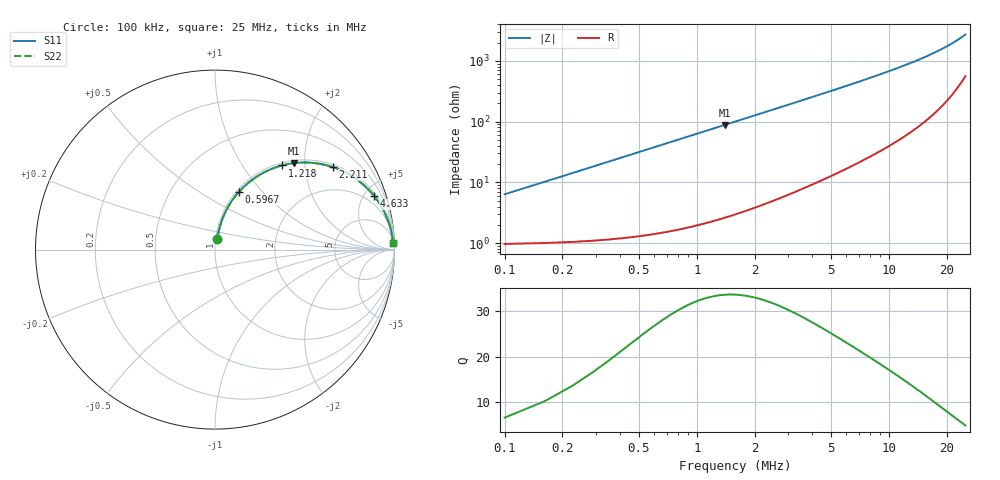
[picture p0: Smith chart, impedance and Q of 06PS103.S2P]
! Coilcraft 0603PS-103 Power Chip Inductor
! 19 February 2003
# MHZ S MA R 50
!Freq  MagS11  AngS11  MagS21  AngS21  MagS12  AngS12  MagS22  AngS22
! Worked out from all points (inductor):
!   403 points, 100 kHz to 25 MHz, reference 50 ohm
!   read as one part in series: L = 10 uH near 224.2 kHz
!   highest Q = 33.7 at 1.404 MHz (marker M1), where L = 10 uH
!   S11 on the Smith chart (normalised r, x): 100 kHz: 1.02, +0.13; 596.7 kHz: 1.03, +0.75; 1.218 MHz: 1.05, +1.53; 2.211 MHz: 1.09, +2.79; 4.633 MHz: 1.23, +5.90; 25 MHz: 12, +53
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0.1  0.06284 77.7  0.9885 -3.6  0.9885 -3.6  0.06284 77.7
0.16209  0.1008 78.6  0.9851 -5.8  0.9851 -5.8  0.1008 78.6
0.28627  0.1755 76.4  0.9739 -10.1  0.9739 -10.1  0.1755 76.4
0.34836  0.2118 74.8  0.9663 -12.2  0.9663 -12.2  0.2118 74.8
0.47254  0.2816 71.2  0.9476 -16.3  0.9476 -16.3  0.2816 71.2
0.59672  0.3471 67.6  0.925 -20.3  0.925 -20.3  0.3471 67.6
0.84508  0.4631 60.6  0.8714 -27.6  0.8714 -27.6  0.4631 60.6
1.03135  0.5367 55.8  0.8274 -32.4  0.8274 -32.4  0.5367 55.8
1.21762  0.5995 51.5  0.7826 -36.8  0.7826 -36.8  0.5995 51.5
1.40389  0.6525 47.6  0.7387 -40.7  0.7387 -40.7  0.6525 47.6
1.77643  0.7347 41.0  0.6568 -47.3  0.6568 -47.3  0.7347 41.0
2.21106  0.801 35.1  0.5746 -53.2  0.5746 -53.2  0.801 35.1
2.64569  0.8462 30.4  0.5066 -57.8  0.5066 -57.8  0.8462 30.4
3.08032  0.8778 26.8  0.4507 -61.3  0.4507 -61.3  0.8778 26.8
4.26003  0.927 20.0  0.3421 -67.9  0.3421 -67.9  0.927 20.0
4.63257  0.9363 18.5  0.317 -69.3  0.317 -69.3  0.9363 18.5
6.37109  0.962 13.5  0.2337 -73.9  0.2337 -73.9  0.962 13.5
8.42006  0.9754 10.1  0.1754 -76.9  0.1754 -76.9  0.9754 10.1
12.58009  0.986 6.4  0.1112 -79.6  0.1112 -79.6  0.986 6.4
16.74012  0.9898 4.3  0.07609 -80.1  0.07609 -80.1  0.9898 4.3
20.90015  0.9913 3.0  0.05307 -79.1  0.05307 -79.1  0.9913 3.0
25  0.9918 2.1  0.03656 -76.1  0.03656 -76.1  0.9918 2.1
